(* Logix 5000 Module export ; software revision 30.00 *)

MODULES
   ISC_CAM : ETHERNET-MODULE (Ethernet 192.168.1.254, rev 1.1, Output RPI 10 ms)
        ISC_CAM:I.DATA[0]   // Status
        ISC_CAM:I.DATA[0].0   // Life_Bit
        ISC_CAM:I.DATA[0].1   // SystemReady
        ISC_CAM:I.DATA[0].4   // Error
        ISC_CAM:I.DATA[0].8   // EncoderStatus
        ISC_CAM:I.DATA[1]   // Fault Code Word 1
        ISC_CAM:I.DATA[1].0   // Line controller PLC indicated the drive motor is running, but the encoder does not detect motion
        ISC_CAM:I.DATA[1].1   // Line controller PLC indicates the drive motor is off, but the encoder detects belt motion
        ISC_CAM:I.DATA[1].2   // Belt detected to move too slow (and not stopped)
        ISC_CAM:I.DATA[1].3   // Belt detected to move too fast
        ISC_CAM:I.DATA[1].4   // Status of photoeye Product Sensor 1
        ISC_CAM:I.DATA[1].5   // Status of photoeye Product Sensor 2 (Optional)
        ISC_CAM:I.DATA[1].6   // Status of photoeye Product Sensor 3 (Optional)
        ISC_CAM:I.DATA[1].7   // Peg sensor blocked continuously with belt moving
        ISC_CAM:I.DATA[1].8   // Peg not seen while expected
        ISC_CAM:I.DATA[1].9   // Gap for next product
        ISC_CAM:I.DATA[1].10   // Too much or too low voltage from power supply
        ISC_CAM:I.DATA[1].11   // Too much or too little current draw (indicates short or cable disconnected)
        ISC_CAM:I.DATA[1].12   // IO-Link error port C0
        ISC_CAM:I.DATA[1].13   // IO-Link error port C1
        ISC_CAM:I.DATA[1].14   // IO-Link error port C2
        ISC_CAM:I.DATA[1].15   // IO-Link error port C3
        ISC_CAM:I.DATA[2]   // Fault Code Word 2
        ISC_CAM:I.DATA[3]   // ProductsOnBelt - Count of current products on the belt (Optional in V1 scope)
        ISC_CAM:I.DATA[4]   // Troughput - Products per time unit on DPE (Optional in V1 scope)
        ISC_CAM:I.DATA[5]   // BeltSpeed - Current speed of the belt
        ISC_CAM:I.DATA[6]   // AccelerationSpeed - Acceleration speed of the belt
        ISC_CAM:I.DATA[7]   // SensorStatus - Active status of all inputs connected
        ISC_CAM:I.DATA[7].0   // Status - 0
        ISC_CAM:I.DATA[7].1   // Product Sensor
        ISC_CAM:I.DATA[7].2   // Peg Sensor Divert 1 (AIM Only)
        ISC_CAM:I.DATA[7].3   // Valve Divert 1
        ISC_CAM:I.DATA[7].4   // Peg Sensor Divert 2 (AIM Only)
        ISC_CAM:I.DATA[7].5   // Valve Divert 2
        ISC_CAM:I.DATA[7].6   // Discrete Divert Signal
        ISC_CAM:I.DATA[7].7   // Run/Error
        ISC_CAM:I.DATA[7].8   // Status - 8
        ISC_CAM:I.DATA[7].9   // Status - 9
        ISC_CAM:I.DATA[7].10   // Status - 10
        ISC_CAM:I.DATA[7].11   // Status - 11
        ISC_CAM:I.DATA[7].12   // Status - 12
        ISC_CAM:I.DATA[7].13   // Status - 13
        ISC_CAM:I.DATA[7].14   // Status - 14
        ISC_CAM:I.DATA[7].15   // Status - 15
        ISC_CAM:I.DATA[9]   // Uptime MSB - Time since the ISC has been booted (sec)
        ISC_CAM:I.DATA[10]   // Uptime LSB - Time since the ISC has been booted (sec)
        ISC_CAM:I.DATA[12]   // Parameter number feedback
        ISC_CAM:I.DATA[13]   // Parameter Status
        ISC_CAM:I.DATA[13].0   // Parameter read succesfully
        ISC_CAM:I.DATA[13].1   // Parameter write succesfully
        ISC_CAM:I.DATA[13].2   // Parameter number not exist or read only
        ISC_CAM:I.DATA[13].3   // Parameter value is out of range
        ISC_CAM:I.DATA[14]   // Parameter data register High Word
        ISC_CAM:I.DATA[15]   // Parameter data register Low Word
        ISC_CAM:I.DATA[16]   // BeltRunTime MSW
        ISC_CAM:I.DATA[17]   // BeltRunTime LSW
        ISC_CAM:I.DATA[18]   // BeltTravelDistance MSW
        ISC_CAM:I.DATA[19]   // BeltTravelDistance LSW
        ISC_CAM:I.DATA[20]   // ActivationCount MSW - Cumulative number of activations divert zone 0
        ISC_CAM:I.DATA[21]   // ActivationCount LSW
        ISC_CAM:I.DATA[22]   // ActivationCount MSW - Cumulative number of activations divert zone 1
        ISC_CAM:I.DATA[23]   // ActivationCount LSW
        ISC_CAM:I.DATA[24]   // ActivationCount MSW - Cumulative number of activations divert zone 2
        ISC_CAM:I.DATA[25]   // ActivationCount LSW
        ISC_CAM:I.DATA[26]   // ProductCount MSW - Cumulative number of products on the belt
        ISC_CAM:I.DATA[27]   // ProductCount LSW
        ISC_CAM:I.DATA[28]   // StartStops MSW - Cumulative number of start stops of the belt
        ISC_CAM:I.DATA[29]   // StartStops LSW
        ISC_CAM:I.DATA[30]   // GapToSmallCount MSW - Cumulative number a too small gap was detected
        ISC_CAM:I.DATA[31]   // GapToSmallCount LSW
        ISC_CAM:I.DATA[32]   // FaultCount
        ISC_CAM:I.DATA[33]   // MaxBeltSpeed
        ISC_CAM:I.DATA[34]   // PeakAcceleration
        ISC_CAM:I.DATA[35]   // PeakDecceleration
        ISC_CAM:O.DATA[0]   // Status
        ISC_CAM:O.DATA[0].0   // Life_Bit
        ISC_CAM:O.DATA[0].1   // BeltRunning
        ISC_CAM:O.DATA[0].7   // Reset_Error
        ISC_CAM:O.DATA[1]   // Divert destination of the next product that will be arriving on the belt
        ISC_CAM:O.DATA[2]   // RunMode
        ISC_CAM:O.DATA[3]   // ProductCountExit0
        ISC_CAM:O.DATA[4]   // ProductCountExit1
        ISC_CAM:O.DATA[5]   // ProductCountExit2
        ISC_CAM:O.DATA[6]   // ProductCountExit3
        ISC_CAM:O.DATA[7]   // DestinationEnableDisable
        ISC_CAM:O.DATA[12]   // Parameter number
        ISC_CAM:O.DATA[13]   // Read/Whrite Parameter
        ISC_CAM:O.DATA[13].0   // Read Parameter
        ISC_CAM:O.DATA[13].1   // Whrite Parameter
        ISC_CAM:O.DATA[14]   // Parameter Data MSW
        ISC_CAM:O.DATA[15]   // Parameter Data MSW
END_MODULES
